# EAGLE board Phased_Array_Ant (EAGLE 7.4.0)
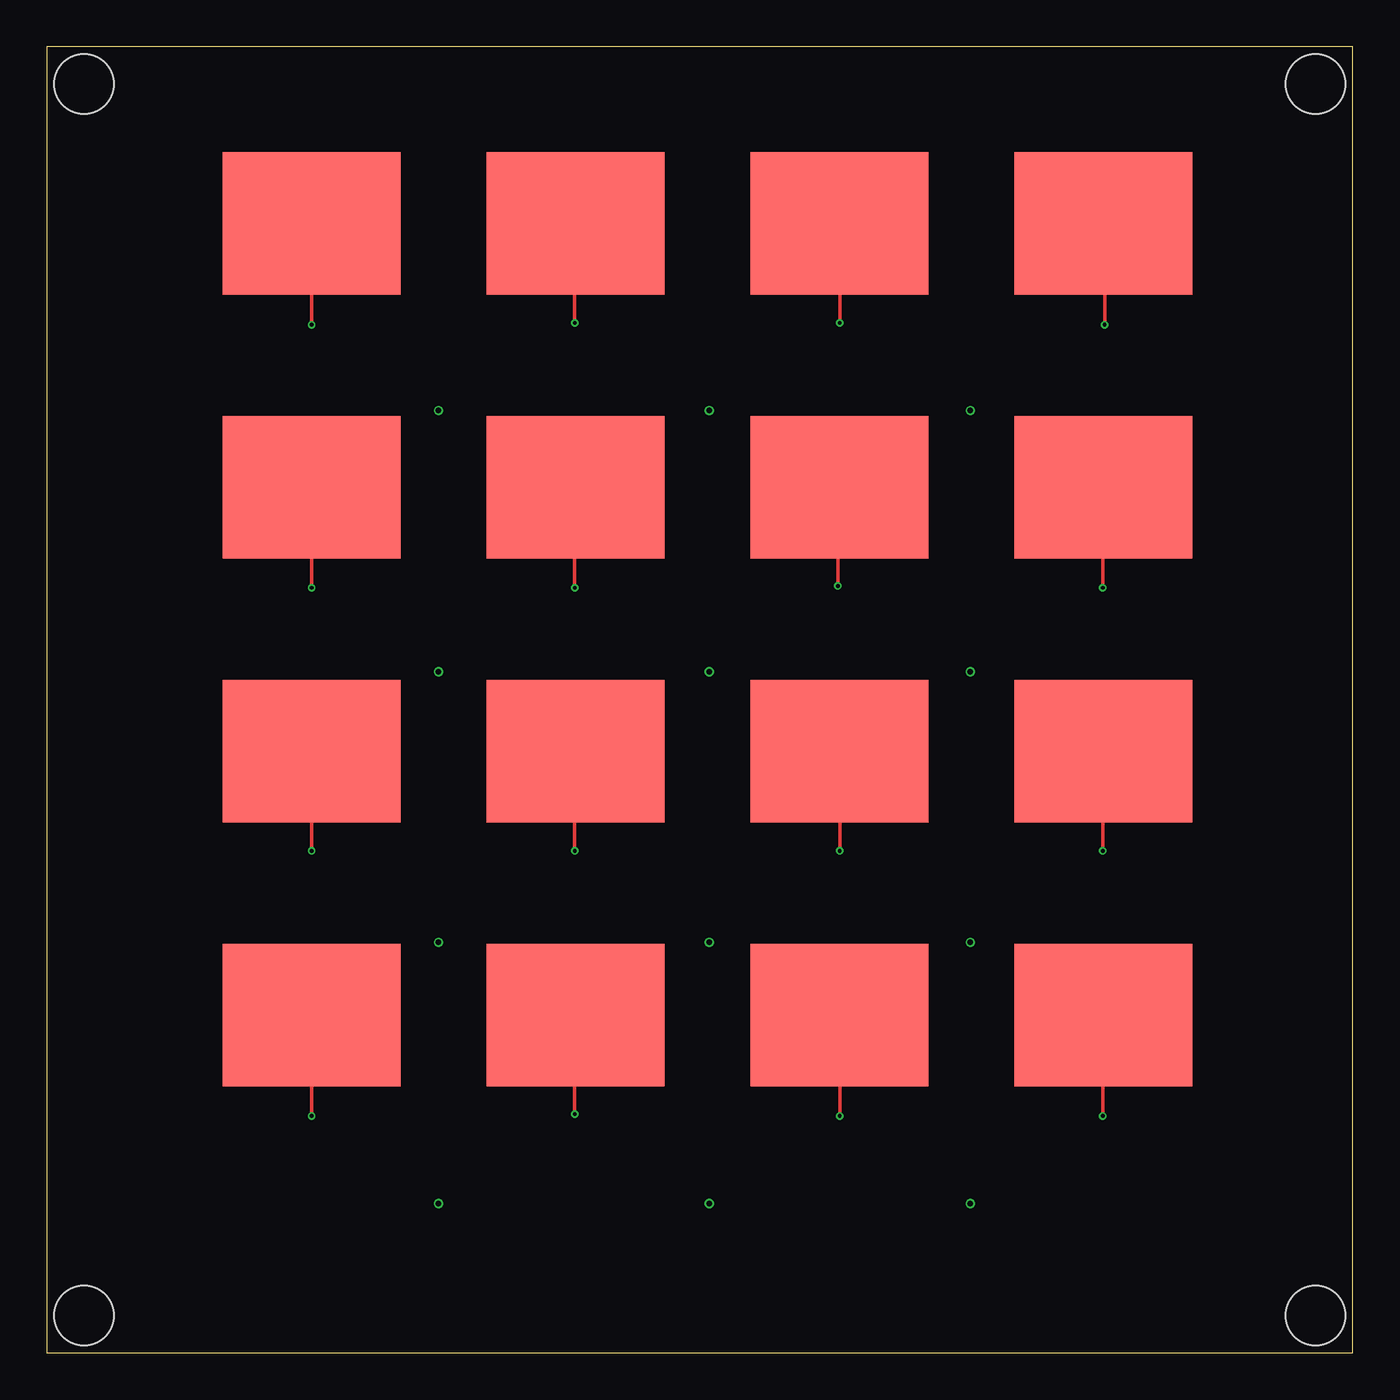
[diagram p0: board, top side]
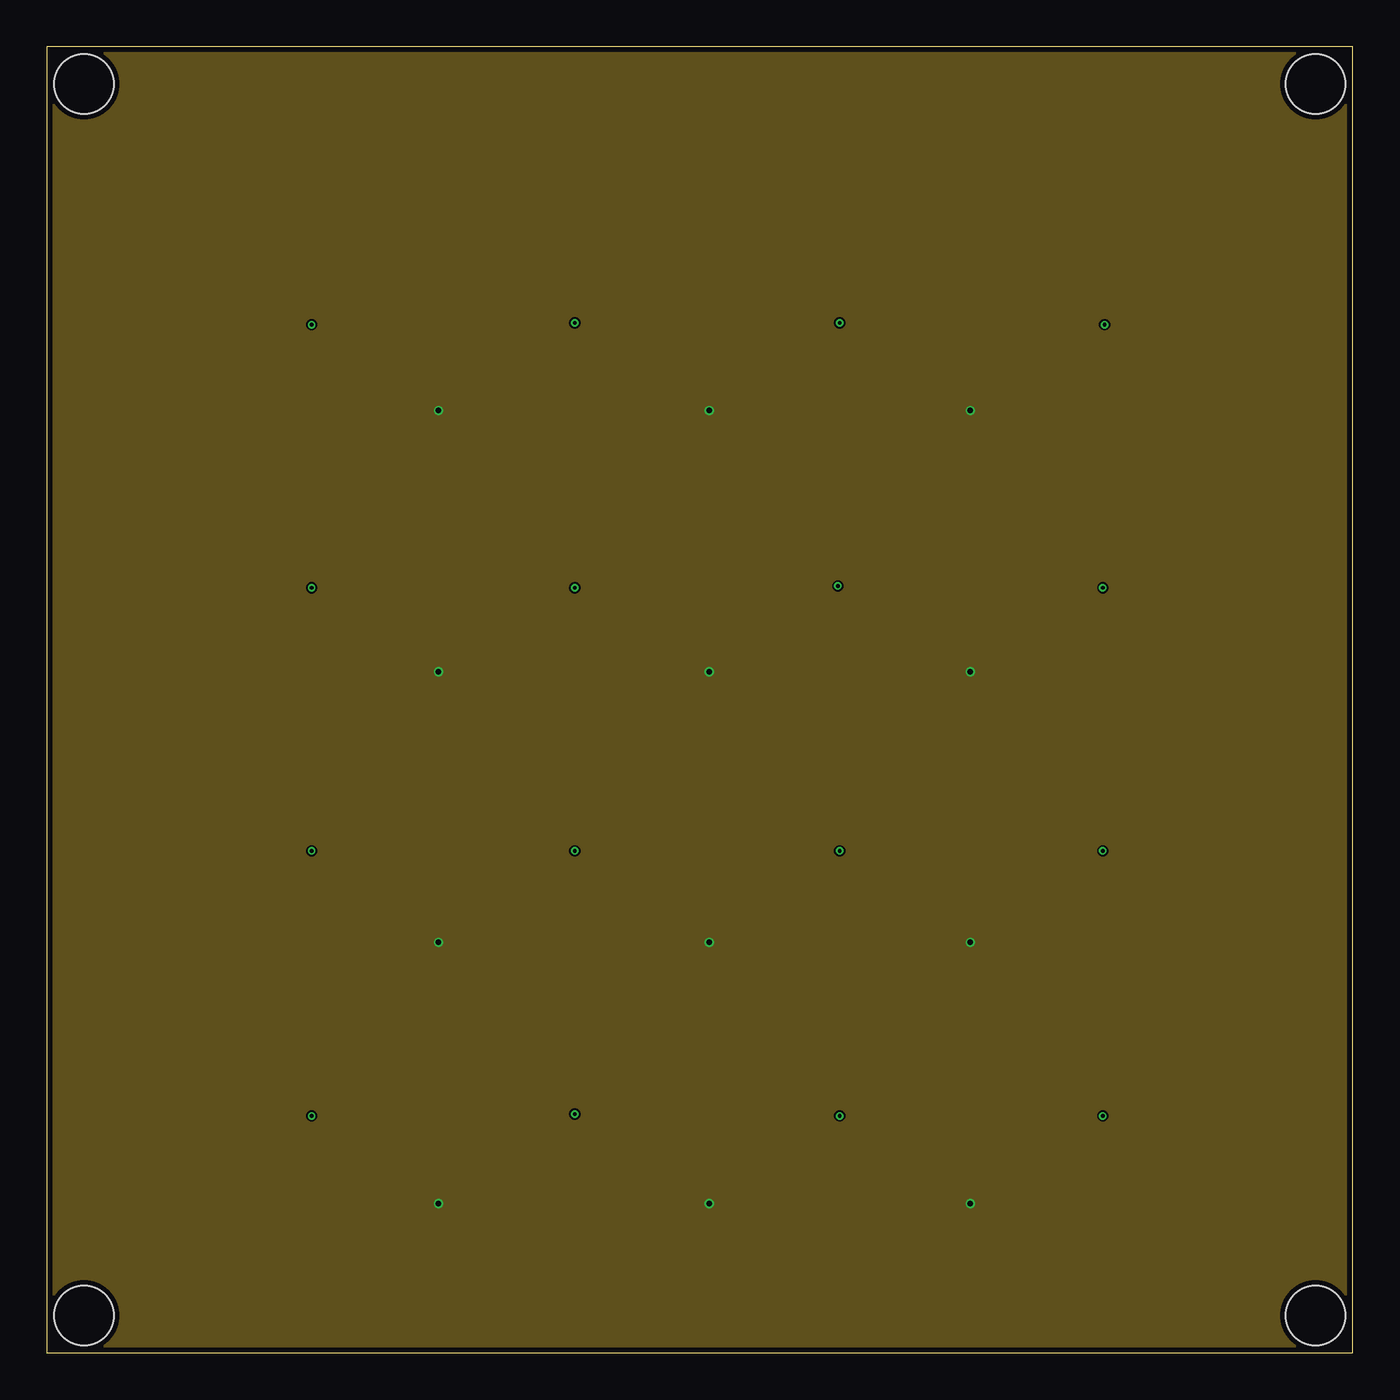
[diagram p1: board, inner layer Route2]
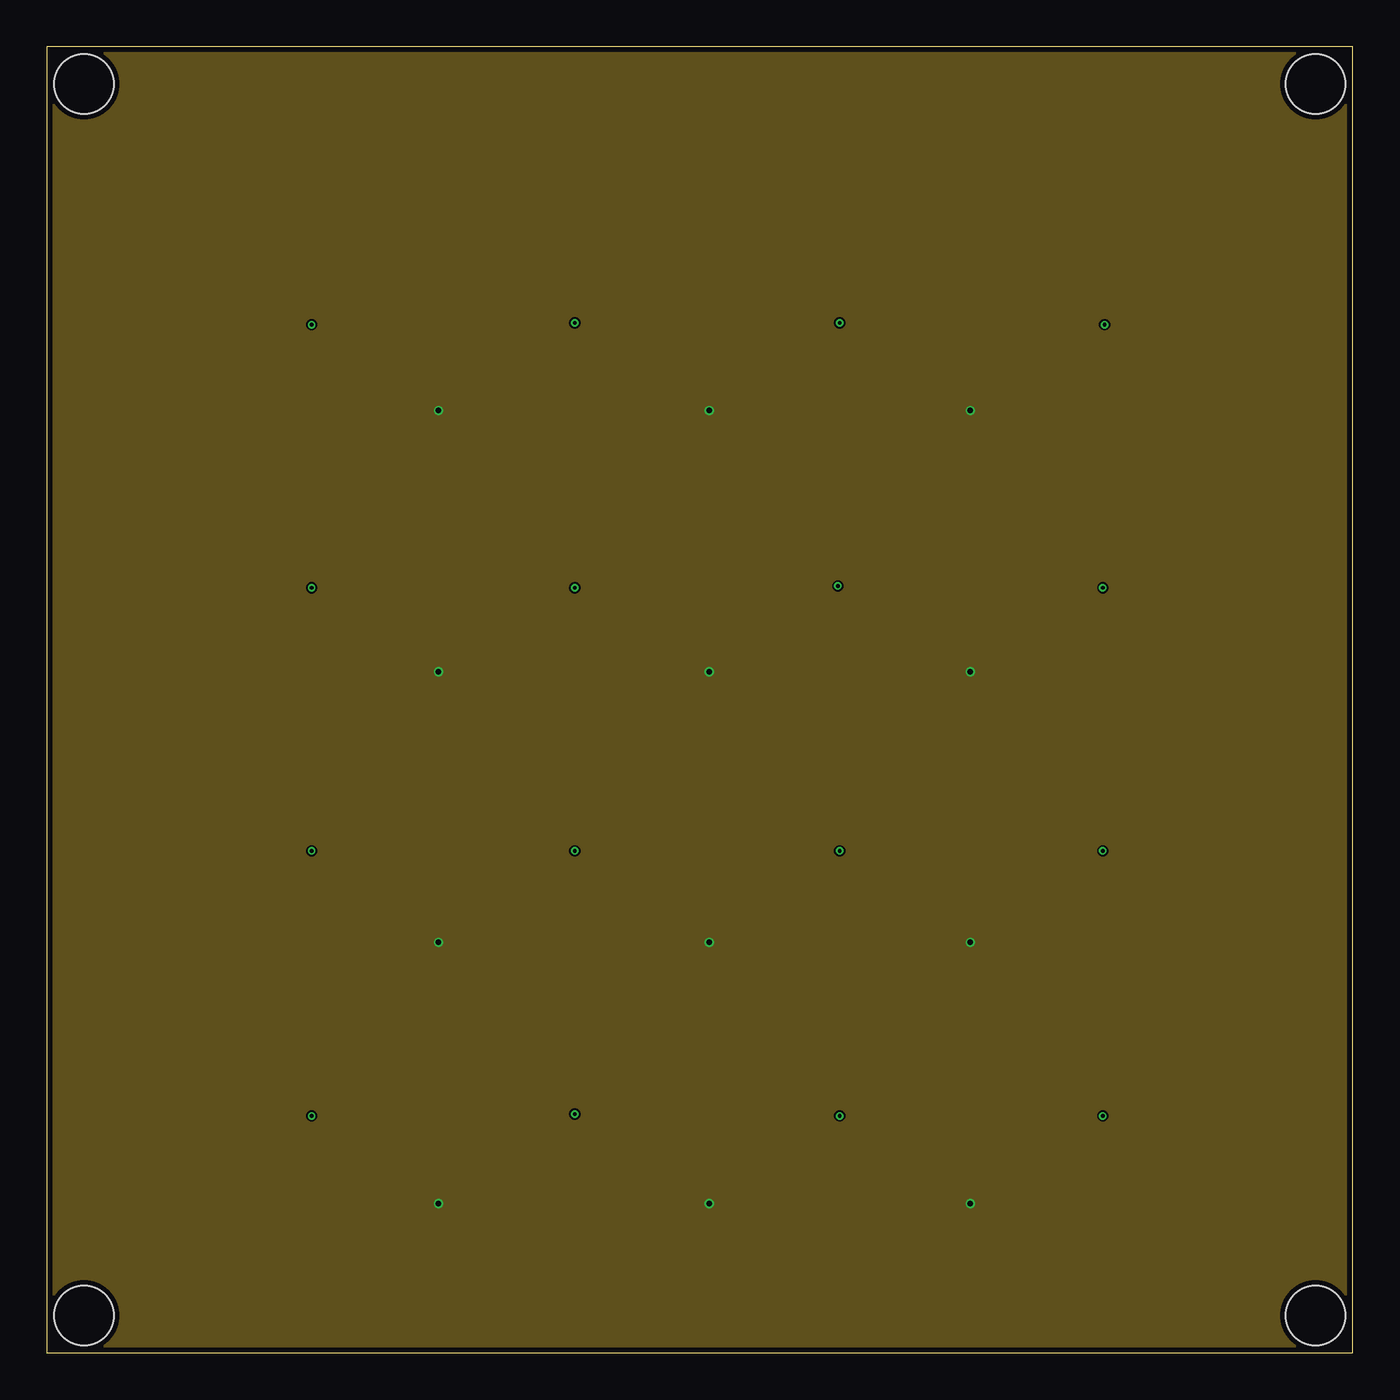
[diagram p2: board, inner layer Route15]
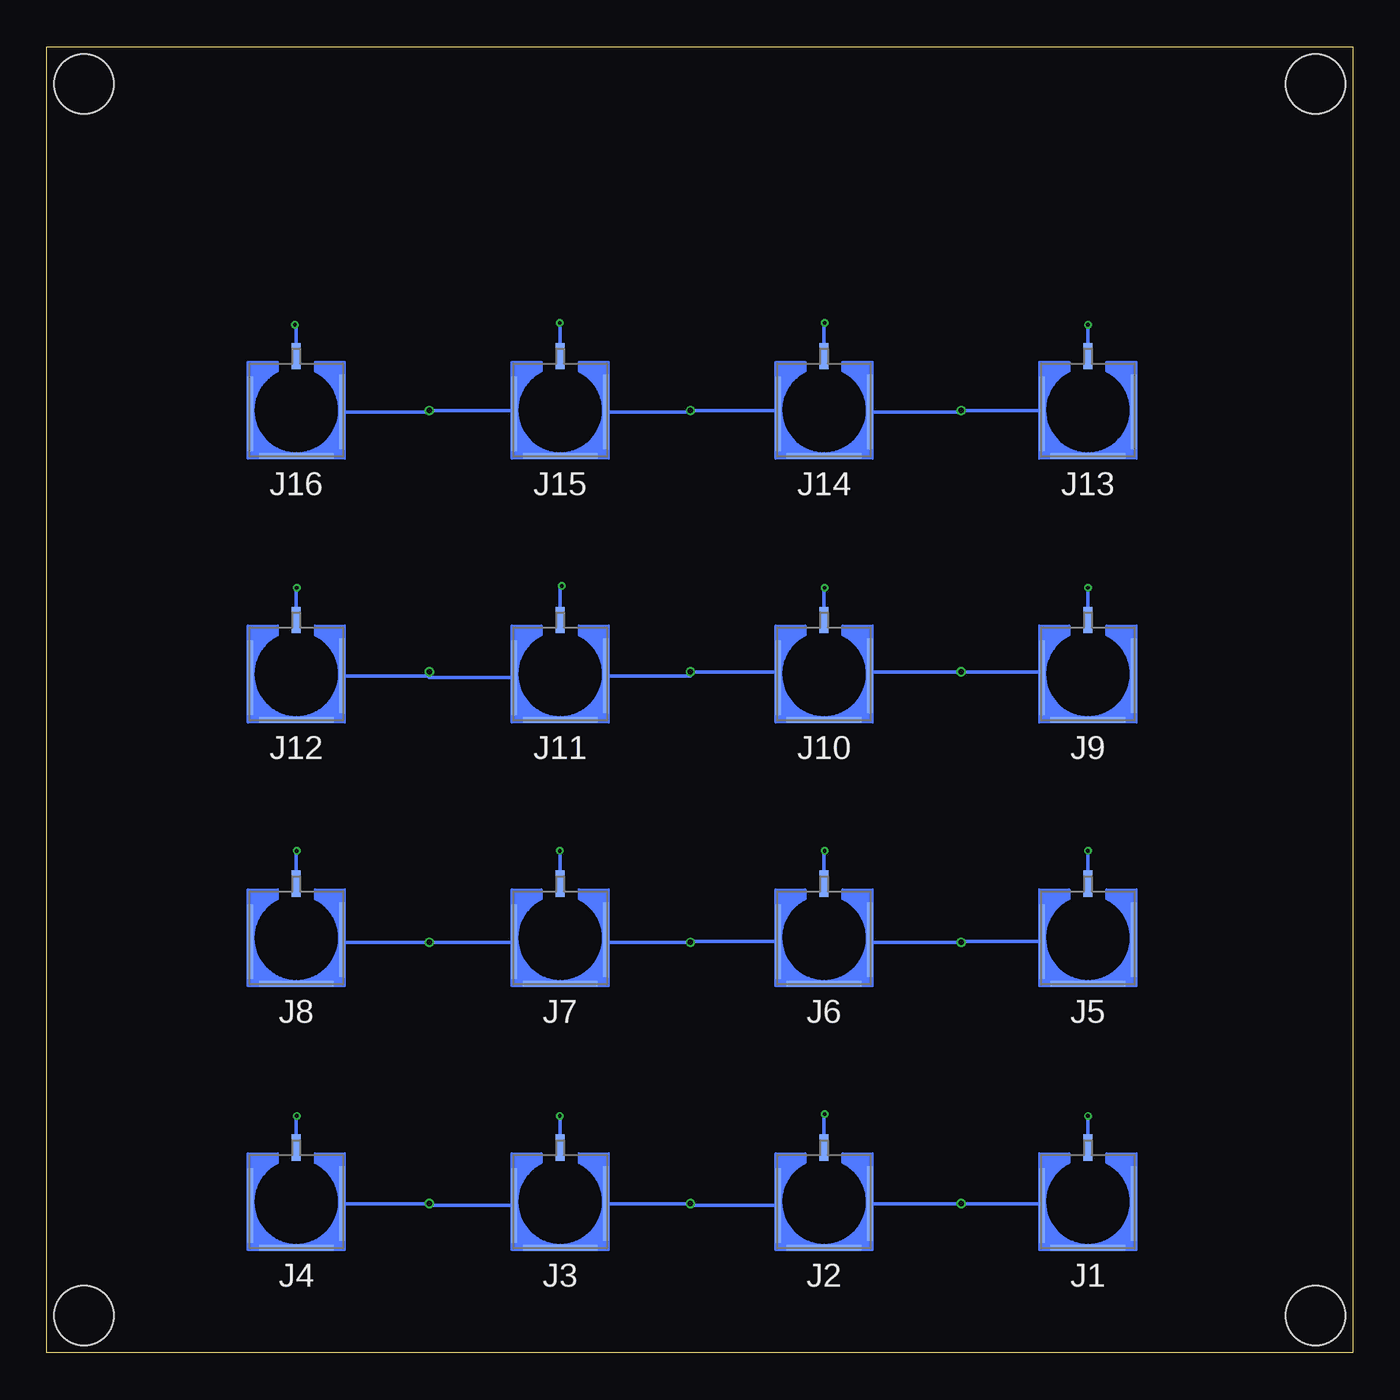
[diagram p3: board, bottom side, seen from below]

Size 70 x 70 mm. Coordinates in mm from the lower left corner, seen from the top.
Outline: 0,0 70,0 70,70 0,70 0,0
Copper layers (1+2*3+14*15+16): Top 0.035mm / dielectric 0.11mm / Route2 0.035mm / dielectric 0.6mm / Route3 0.035mm / dielectric 0.11mm / Route14 0.035mm / dielectric 0.6mm / Route15 0.035mm / dielectric 0.11mm / Bottom 0.035mm
Design rules "PCBWay_6L_100um-Track": minimum track width 0.1mm, minimum drill 0.3mm, track to track 0.1mm, track to pad 0.1mm, pad to pad 0.1mm, via to via 0.1mm, smd to smd 0mil, copper to edge 0.3mm, drill to drill 10mil, minimum pad ring 6mil, minimum via ring 0.1mm, stop-mask expansion 2mil, vias tented up to drill 0.45mm, thermal gap 0.2mm
Holes 3.2 mm at 2,2 68,2 68,68 2,68

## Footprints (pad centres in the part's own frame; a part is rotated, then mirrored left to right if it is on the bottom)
60124102122403 = smd 0.48 x 1.4: 1 0,-2.9 | smd 0.3 x 4: 2 -2.45,0.1; 4 2.45,0.2 | smd 4 x 0.3: 3 0,2.45
10.5GHZ_ANT = smd 9.538 x 7.636: P$1 0,0

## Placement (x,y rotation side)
J1  4_1  [60124102122403]  14.2,8.1 180 bottom
J2  4_2  [60124102122403]  28.34,8.1 180 bottom
J3  4_3  [60124102122403]  42.48,8.1 180 bottom
J4  4_4  [60124102122403]  56.62,8.1 180 bottom
J5  3_1  [60124102122403]  14.2,22.24 180 bottom
J6  3_2  [60124102122403]  28.34,22.24 180 bottom
J7  3_3  [60124102122403]  42.48,22.24 180 bottom
J8  3_4  [60124102122403]  56.62,22.24 180 bottom
J9  2_1  [60124102122403]  14.2,36.38 180 bottom
J10  2_2  [60124102122403]  28.34,36.38 180 bottom
J11  2_3  [60124102122403]  42.48,36.38 180 bottom
J12  2_4  [60124102122403]  56.62,36.38 180 bottom
J13  1_1  [60124102122403]  14.2,50.52 180 bottom
J14  1_2  [60124102122403]  28.34,50.52 180 bottom
J15  1_3  [60124102122403]  42.48,50.52 180 bottom
J16  1_4  [60124102122403]  56.62,50.52 180 bottom
U$1  10.5GHZ_ANT  [10.5GHZ_ANT]  14.2,18.1 0 top
U$2  10.5GHZ_ANT  [10.5GHZ_ANT]  28.34,18.1 0 top
U$3  10.5GHZ_ANT  [10.5GHZ_ANT]  42.48,18.1 0 top
U$4  10.5GHZ_ANT  [10.5GHZ_ANT]  56.62,18.1 0 top
U$5  10.5GHZ_ANT  [10.5GHZ_ANT]  14.2,32.24 0 top
U$6  10.5GHZ_ANT  [10.5GHZ_ANT]  28.34,32.24 0 top
U$7  10.5GHZ_ANT  [10.5GHZ_ANT]  42.48,32.24 0 top
U$8  10.5GHZ_ANT  [10.5GHZ_ANT]  56.62,32.24 0 top
U$9  10.5GHZ_ANT  [10.5GHZ_ANT]  14.2,46.38 0 top
U$10  10.5GHZ_ANT  [10.5GHZ_ANT]  28.34,46.38 0 top
U$11  10.5GHZ_ANT  [10.5GHZ_ANT]  42.48,46.38 0 top
U$12  10.5GHZ_ANT  [10.5GHZ_ANT]  56.62,46.38 0 top
U$13  10.5GHZ_ANT  [10.5GHZ_ANT]  14.2,60.52 0 top
U$14  10.5GHZ_ANT  [10.5GHZ_ANT]  28.34,60.52 0 top
U$15  10.5GHZ_ANT  [10.5GHZ_ANT]  42.48,60.52 0 top
U$16  10.5GHZ_ANT  [10.5GHZ_ANT]  56.62,60.52 0 top

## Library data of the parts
J1-J16 = Eagle_WR-SMP_rev21a; DATASHEET-URL: https://www.we-online.com/catalog/datasheet/60124102122403.pdf; GENDER: Plug; INTERFACE: MIL-STD-348; MOUNT: SMT; ORIENTATION-TYPE: Straight; PART-NUMBER: 60124102122403; Z: 50Ohm
U$1-U$16 = My_Library_RADAR

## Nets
GND: J1.2 J1.3 J1.4 J2.2 J2.3 J2.4 J3.2 J3.3 J3.4 J4.2 J4.3 J4.4 J5.2 J5.3 J5.4 J6.2 J6.3 J6.4 J7.2 J7.3 J7.4 J8.2 J8.3 J8.4 J9.2 J9.3 J9.4 J10.2 J10.3 J10.4 J11.2 J11.3 J11.4 J12.2 J12.3 J12.4 J13.2 J13.3 J13.4 J14.2 J14.3 J14.4 J15.2 J15.3 J15.4 J16.2 J16.3 J16.4
N$1: J1.1 U$1.P$1
N$2: J2.1 U$2.P$1
N$3: J3.1 U$3.P$1
N$4: J4.1 U$4.P$1
N$5: J5.1 U$5.P$1
N$6: J6.1 U$6.P$1
N$7: J7.1 U$7.P$1
N$8: J8.1 U$8.P$1
N$9: J9.1 U$9.P$1
N$10: J10.1 U$10.P$1
N$11: J11.1 U$11.P$1
N$12: J12.1 U$12.P$1
N$13: J13.1 U$13.P$1
N$14: J14.1 U$14.P$1
N$15: J15.1 U$15.P$1
N$16: J16.1 U$16.P$1

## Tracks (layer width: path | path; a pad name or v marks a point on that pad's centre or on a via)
GND  (via drill 0.3)
  Bottom 0.2: J1.4 16.65,8 v21,8 J2.2 | J13.4 16.65,50.5 v21,50.5 21,50.42 J14.2 | J14.4 30.79,50.5 v35.5,50.5 35.5,50.42 J15.2 | J16.2 49.5,50.42 v49.5,50.5 44.93,50.5 J15.4 | J9.4 16.65,36.5 v21,36.5 25.89,36.5 J10.2 | J10.4 30.79,36.5 v35.5,36.5 35.5,36.28 J11.2 | J12.2 49.5,36.28 v49.5,36.5 49.5,36.18 J11.4 | J8.2 54.17,22 v49.5,22 44.93,22 J7.4 | J7.2 40.03,22 v35.5,22 35.5,22.04 J6.4 | J5.4 21,22.04 v21,22 25.89,22 J6.2 | J2.4 35.5,7.9 v35.5,8 J3.2 | J3.4 49.5,7.9 v49.5,8 J4.2
  pour Route2: 0,70 70,70 70,0 0,0
  pour Route15: 0,70 70,70 70,0 0,0
N$1  (via drill 0.2)
  Top 0.2: v14.2,12.7 U$1.P$1
  Bottom 0.2: J1.1 v14.2,12.7
N$2  (via drill 0.2)
  Top 0.2: v28.3,12.8 28.3,18.1 U$2.P$1
  Bottom 0.2: J2.1 28.34,12.8 v28.3,12.8
N$3  (via drill 0.2)
  Top 0.2: v42.5,12.7 42.5,18.1 U$3.P$1
  Bottom 0.2: J3.1 42.48,12.7 v42.5,12.7
N$4  (via drill 0.2)
  Top 0.2: v56.6,12.7 56.6,18.1 U$4.P$1
  Bottom 0.2: J4.1 56.62,12.7 v56.6,12.7
N$5  (via drill 0.2)
  Top 0.2: v14.2,26.9 U$5.P$1
  Bottom 0.2: J5.1 v14.2,26.9
N$6  (via drill 0.2)
  Top 0.2: v28.3,26.9 28.3,32.24 U$6.P$1
  Bottom 0.2: J6.1 28.34,26.9 v28.3,26.9
N$7  (via drill 0.2)
  Top 0.2: v42.5,26.9 42.5,32.24 U$7.P$1
  Bottom 0.2: J7.1 42.48,26.9 v42.5,26.9
N$8  (via drill 0.2)
  Top 0.2: v56.6,26.9 56.6,32.24 U$8.P$1
  Bottom 0.2: J8.1 56.62,26.9 v56.6,26.9
N$9  (via drill 0.2)
  Top 0.2: v14.2,41 U$9.P$1
  Bottom 0.2: J9.1 v14.2,41
N$10  (via drill 0.2)
  Top 0.2: v28.3,41 28.3,46.38 U$10.P$1
  Bottom 0.2: J10.1 28.34,41 v28.3,41
N$11  (via drill 0.2)
  Top 0.2: v42.4,41.1 42.4,46.38 U$11.P$1
  Bottom 0.2: J11.1 42.48,41.1 v42.4,41.1
N$12  (via drill 0.2)
  Top 0.2: v56.6,41 56.6,46.38 U$12.P$1
  Bottom 0.2: J12.1 56.62,41 v56.6,41
N$13  (via drill 0.2)
  Top 0.2: v14.2,55.1 U$13.P$1
  Bottom 0.2: J13.1 v14.2,55.1
N$14  (via drill 0.2)
  Top 0.2: v28.3,55.2 28.3,60.52 U$14.P$1
  Bottom 0.2: J14.1 28.34,55.2 v28.3,55.2
N$15  (via drill 0.2)
  Top 0.2: v42.5,55.2 42.5,60.52 U$15.P$1
  Bottom 0.2: J15.1 42.48,55.2 v42.5,55.2
N$16  (via drill 0.2)
  Top 0.2: v56.7,55.1 56.7,60.52 U$16.P$1
  Bottom 0.2: J16.1 56.62,55.1 v56.7,55.1

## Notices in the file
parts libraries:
Eagle_WR-SMP_rev21a: Copyright: Würth Elektronik
